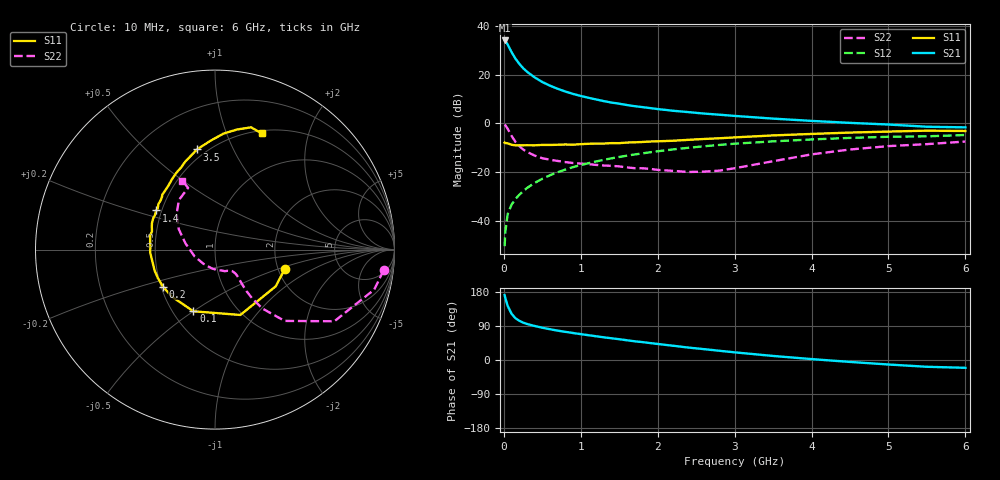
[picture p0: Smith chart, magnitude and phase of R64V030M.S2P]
! SIEMENS Small Signal Semiconductors
! BFR193
! Si NPN RF Bipolar Junction Transistor in SOT23
! VCE = 4 V  IC = 30 mA
! Common Emitter S-Parameters:  May  1996
# GHz  S  MA  R  50
!  f  S11  S21  S12  S22
! GHz  MAG  ANG  MAG  ANG  MAG  ANG  MAG  ANG
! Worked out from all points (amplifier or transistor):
!   36 points, 10 MHz to 6 GHz, reference 50 ohm
!   highest |S21| = 34.1 dB at 10 MHz (marker M1)
!   |S21| within 3 dB of that: start of sweep to 71.69 MHz
!   unconditionally stable (mu >= 1): 477.7 MHz to 1.881 GHz; 1.977 GHz to 2.012 GHz
!   at 250 MHz: K = 0.90, MSG = 25.3 dB, |S12| = -27.9 dB
!   at 1.4 GHz: K = 1.02, MAG = 10.6 dB, |S12| = -14.3 dB
!   at 6 GHz: K = 0.95, MSG = 1.6 dB, |S12| = -4.8 dB
!   lowest NFmin = 1.90 dB at 450 MHz
!   S11 on the Smith chart (normalised r, x): 10 MHz: 2.17, -0.57; 100 MHz: 0.63, -0.50; 200 MHz: 0.51, -0.24; 1.4 GHz: 0.47, +0.24; 3.5 GHz: 0.45, +0.73; 6 GHz: 0.53, +1.34
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0.01  0.4033 -15.7  50.73 171.2  0.003 85.6  0.9467 -7.0
0.02  0.3953 -31.2  49.33 162.9  0.006 81.2  0.9146 -14.1
0.05  0.3906 -68.8  41.94 142.6  0.0137 71.1  0.7755 -31.0
0.1  0.3642 -109.3  29.34 122.1  0.0214 66.2  0.5551 -45.7
0.15  0.3554 -132.1  21.57 110.4  0.0278 66.0  0.4209 -51.2
0.2  0.3561 -144.7  16.86 103.6  0.0341 67.8  0.3427 -52.7
0.25  0.3556 -153.5  13.71 98.7  0.0403 68.4  0.2922 -52.8
0.3  0.3563 -160.9  11.59 95.1  0.0469 70.3  0.2599 -52.3
0.4  0.3554 -170.1  8.84 89.8  0.0598 71.3  0.2184 -51.0
0.5  0.3617 -177.7  7.098 85.2  0.0727 71.9  0.1925 -49.8
0.6  0.3606 177.5  5.968 81.2  0.086 71.5  0.1796 -49.5
0.7  0.3647 172.6  5.15 77.5  0.0992 71.1  0.1694 -49.8
0.8  0.3694 167.7  4.522 74.3  0.1127 70.0  0.1604 -50.6
0.9  0.3656 163.7  4.039 71.2  0.1264 69.2  0.1535 -51.3
1.1  0.3814 157.0  3.367 65.4  0.1524 67.3  0.1457 -55.5
1.4  0.3937 146.3  2.685 57.3  0.1917 63.5  0.1343 -62.9
1.7  0.4088 137.8  2.261 49.4  0.2303 59.4  0.1202 -73.7
2.2  0.4405 126.2  1.822 37.6  0.2923 52.2  0.106 -100.4
3.5  0.567 100.2  1.256 10.7  0.4281 32.2  0.1671 168.5
4.5  0.6487 85.7  1.027 -5.1  0.5043 18.1  0.2912 137.2
5.5  0.7103 73.6  0.855 -17.9  0.5429 4.1  0.3755 113.5
6  0.6982 68.2  0.83 -20.6  0.5783 0.0  0.4242 115.4
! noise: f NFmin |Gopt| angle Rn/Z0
0.45  1.9  0.4  180  0.09
0.9  1.95  0.43  -173  0.11
1.8  2.4  0.58  -144  0.24
